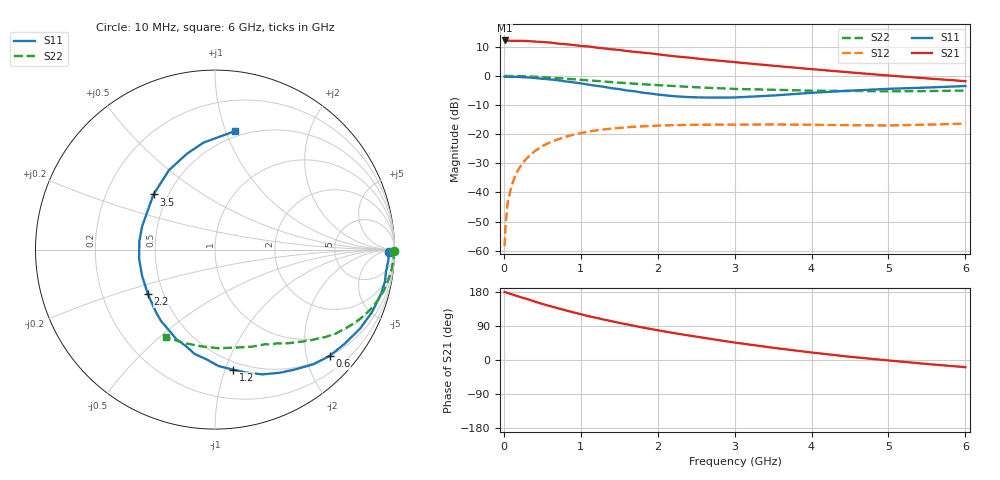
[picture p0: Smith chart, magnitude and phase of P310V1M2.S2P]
! SIEMENS Small Signal Semiconductors
! BFP181
! Si NPN RF Bipolar Junction Transistor in SOT143
! VCE = 10 V  IC = 1.2 mA
! Common Emitter S-Parameters:  March  1996
# GHz  S  MA  R  50
!  f  S11  S21  S12  S22
! GHz  MAG  ANG  MAG  ANG  MAG  ANG  MAG  ANG
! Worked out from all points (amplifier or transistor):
!   36 points, 10 MHz to 6 GHz, reference 50 ohm
!   highest |S21| = 12.1 dB at 10 MHz (marker M1)
!   |S21| within 3 dB of that: start of sweep to 1.393 GHz
!   unconditionally stable (mu >= 1): 3.029 GHz to end of sweep
!   at 250 MHz: K = 0.11, MSG = 20.9 dB, |S12| = -29.8 dB
!   at 1.4 GHz: K = 0.51, MSG = 13.6 dB, |S12| = -18.1 dB
!   at 6 GHz: K = 1.25, MAG = 4.3 dB, |S12| = -16.4 dB
!   S11 on the Smith chart (normalised r, x): 10 MHz: 51, -22; 600 MHz: 0.50, -2.46; 1.2 GHz: 0.43, -1.07; 2.2 GHz: 0.41, -0.26; 3.5 GHz: 0.42, +0.32; 6 GHz: 0.45, +1.08
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0.01  0.9674 -0.8  4.048 179.3  0.0012 70.1  0.9969 -0.3
0.02  0.9672 -1.8  4.031 179.1  0.0025 87.2  0.9937 -0.7
0.05  0.968 -3.5  4.018 176.8  0.0068 88.3  0.9946 -1.8
0.1  0.9607 -7.3  3.993 173.6  0.0129 84.1  0.9969 -3.5
0.15  0.9635 -10.9  3.982 170.3  0.0198 81.4  0.9911 -5.2
0.25  0.9479 -18.2  3.975 163.8  0.0325 77.4  0.9839 -8.7
0.3  0.9417 -21.7  3.957 161.2  0.0388 75.5  0.9785 -10.3
0.4  0.9201 -28.7  3.879 154.3  0.051 71.2  0.9678 -13.7
0.6  0.8709 -42.9  3.735 142.3  0.0724 62.1  0.9349 -20.0
0.8  0.8044 -56.0  3.496 131.2  0.0898 54.0  0.8964 -25.4
1.1  0.7072 -75.7  3.193 115.7  0.1107 44.0  0.8372 -32.5
1.2  0.676 -81.4  3.063 111.3  0.116 40.5  0.8199 -34.8
1.5  0.5923 -101.1  2.786 98.0  0.1279 33.1  0.7637 -40.2
1.8  0.5156 -120.3  2.506 85.8  0.1363 27.0  0.7199 -44.9
2.2  0.449 -146.3  2.179 71.4  0.1426 19.7  0.6704 -50.9
2.4  0.4319 -160.2  2.06 64.8  0.1443 16.9  0.6492 -53.7
2.8  0.4241 174.0  1.82 52.1  0.1457 12.1  0.6142 -59.2
3.5  0.4603 138.1  1.493 32.3  0.1468 6.0  0.5778 -69.5
4  0.5117 120.0  1.305 19.8  0.1447 3.4  0.5577 -78.2
4.5  0.557 106.2  1.147 8.5  0.1426 1.3  0.5501 -87.9
5.5  0.6302 87.5  0.905 -10.5  0.1455 2.2  0.5482 -108.2
6  0.6695 80.5  0.812 -18.9  0.1516 2.0  0.5593 -118.9
